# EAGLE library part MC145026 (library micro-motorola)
ENCODER
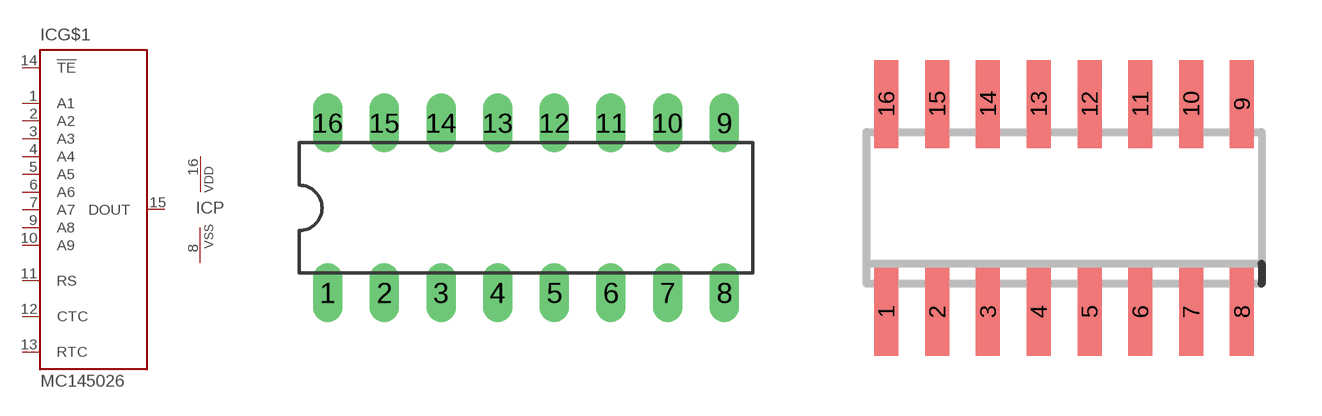
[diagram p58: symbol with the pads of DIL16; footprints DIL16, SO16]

Designator prefix IC; gates G$1=MC145026 P=VSSVDD

## MC145026P (OC_FARNELL: unknown; OC_NEWARK: unknown)  [DIL16]
1  G$1:A1  in
2  G$1:A2  in
3  G$1:A3  in
4  G$1:A4  in
5  G$1:A5  in
6  G$1:A6  in
7  G$1:A7  in
8  P:VSS  pwr
9  G$1:A8  in
10  G$1:A9  in
11  G$1:RS  pas
12  G$1:CTC  pas
13  G$1:RTC  pas
14  G$1:!TE  in
15  G$1:DOUT  in
16  P:VDD  pwr

## MC145026D (OC_FARNELL: unknown; OC_NEWARK: unknown)  [SO16]
Pads as for DIL16

## Footprint DIL16 (pad centres in mm)
Dual In Line Package
drill 0.813 long: 1 -8.89,-3.81; 2 -6.35,-3.81; 3 -3.81,-3.81; 4 -1.27,-3.81; 5 1.27,-3.81; 6 3.81,-3.81; 7 6.35,-3.81; 8 8.89,-3.81; 9 8.89,3.81; 10 6.35,3.81; 11 3.81,3.81; 12 1.27,3.81; 13 -1.27,3.81; 14 -3.81,3.81; 15 -6.35,3.81; 16 -8.89,3.81

## Footprint SO16 (pad centres in mm)
SMALL OUTLINE INTEGRATED CIRCUIT body 3.9 mm/JEDEC MS-012AC
smd 0.6 x 2.2: 1 -4.445,-2.6; 2 -3.175,-2.6; 3 -1.905,-2.6; 4 -0.635,-2.6; 5 0.635,-2.6; 6 1.905,-2.6; 7 3.175,-2.6; 8 4.445,-2.6; 9 4.445,2.6; 10 3.175,2.6; 11 1.905,2.6; 12 0.635,2.6; 13 -0.635,2.6; 14 -1.905,2.6; 15 -3.175,2.6; 16 -4.445,2.6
